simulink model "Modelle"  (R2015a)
settings: Solver=ode45  StartTime=0.0  StopTime=20  FixedStep=0.001  RelTol=1e-4
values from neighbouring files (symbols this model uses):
  A = [    [initLinear.m]    (also in Aufgabe_VglEigenwerte.m = initLinear( l, mp, ms, 0, 0, g, pi ); Versuch2.m = initLinear( l, mp, ms, 0, 0, g, pi ); linPendelZR.m = 1/n *     [ 0   n   0            0   ;                      ; linPendelZR2.m = [0, 1, 0, 0)
  AP = pi    (= 3.14159265359)    [Versuch1.m]    (also in Versuch2.m = 0; Versuch3.m = 0; simGUI.m = 0; Versuch4.m = 0)
  B = [0; 4; 0; 6/l]/(4*ms+mp)    [initLinear.m]    (also in linPendelZR.m = [0 a/n 0 b/n]'; linPendelZR2.m = [0)
  C = [1, 0, 0, 0    [initLinear.m]    (also in linPendelZR.m = [1 0 0 0; 0 0 1 0]')
  D = [0; 0]    [initLinear.m]    (also in linPendelZR.m = [0 0]')
  g = 9.81    [initModell.m]    (also in sFunModell.m = block.DialogPrm(6).Data; para.m; systemPendel_V3.m = stPendel.g; RandwertproblemDGL.m = stPendel.g)
  l = 0.41    [initModell.m]    (also in sFunModell.m = block.DialogPrm(5).Data; para.m; animierePendel.m = stPendel.lPendel; systemPendel_V3.m = stPendel.lPendel)
  mp = 0.177    [initModell.m]    (also in sFunModell.m = block.DialogPrm(3).Data; para.m; systemPendel_V3.m = stPendel.mPendel)
  ms = 7.055    [initModell.m]    (also in sFunModell.m = block.DialogPrm(1).Data; para.m; systemPendel_V3.m = stPendel.mSchlitten)
  Rp = 5.1e-3    (= 0.0051)    [initModell.m]    (also in sFunModell.m = block.DialogPrm(4).Data; para.m)
  Rs = 1.4    [initModell.m]    (also in sFunModell.m = block.DialogPrm(2).Data; para.m)
  teil = 1    [Versuch1.m]    (also in Versuch2.m = 4)
libraries: simulink x2

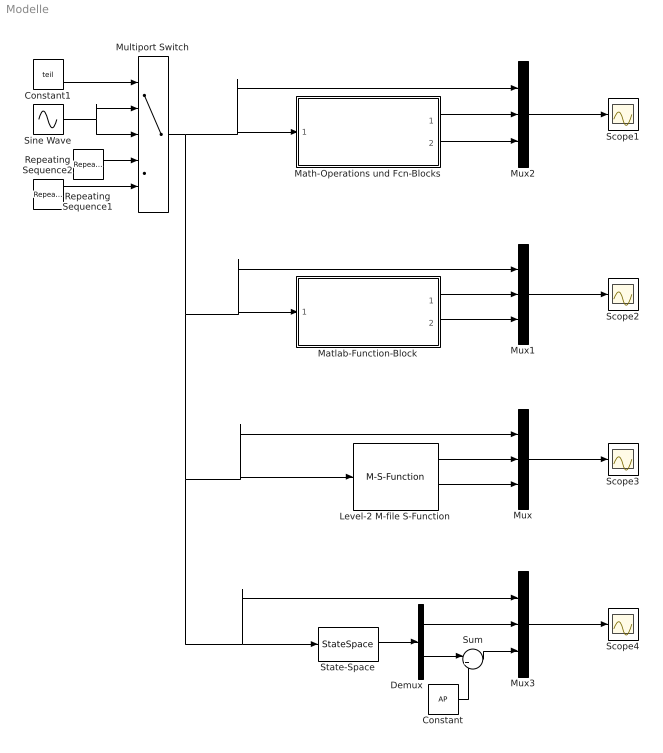
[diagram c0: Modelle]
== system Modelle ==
  Constant : Constant  Value=AP
  Constant1 : Constant  Value=teil
  Demux : Demux  Outputs=2
  Level-2 M-file S-Function : M-S-Function  FunctionName=sFunModell  Parameters=ms, Rs, mp, Rp, l, g, AP
  Math-Operations und Fcn-Blocks : Subsystem
  Matlab-Function-Block : Subsystem
  Multiport Switch : MultiPortSwitch  Inputs=4
  Mux{,1..3} (4 alike) : Mux  Inputs=3
  Repeating Sequence1 : simulink/Sources/Repeating Sequence  rep_seq_t=[0 0.5 0.5001 1.5 1.5001 2]  rep_seq_y=[40 40 -40 -40 40 40]
  Repeating Sequence2 : simulink/Sources/Repeating Sequence  rep_seq_t=[0 1 1.001 2 2.001]  rep_seq_y=[-40 -40 40 40 -40]
  Scope{1..4} (4 alike) : Scope
  Sine Wave : Sin  SampleTime=0
  State-Space : StateSpace  A=A  B=B  C=C  D=D  X0=[0 0 0 0]
  Sum : Sum  Inputs=|++
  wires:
  Math-Operations und Fcn-Blocks/1(xs) -> Mux2/2
  Math-Operations und Fcn-Blocks/2(phi) -> Mux2/3
  Matlab-Function-Block/1(xs) -> Mux1/2
  Matlab-Function-Block/2(phi) -> Mux1/3
  Level-2 M-file S-Function/1 -> Mux/2
  Level-2 M-file S-Function/2 -> Mux/3
  State-Space/1 -> Demux/1
  Demux/1 -> Mux3/2
  Multiport Switch/1 -> Level-2 M-file S-Function/1, Mux/1, Mux3/1, State-Space/1, Matlab-Function-Block/1(F), Mux1/1, Math-Operations und Fcn-Blocks/1(F), Mux2/1
  Mux2/1 -> Scope1/1
  Mux1/1 -> Scope2/1
  Mux3/1 -> Scope4/1
  Mux/1 -> Scope3/1
  Constant1/1 -> Multiport Switch/1
  Sine Wave/1 -> Multiport Switch/2, Multiport Switch/3
  Repeating Sequence1/1 -> Multiport Switch/4
  Repeating Sequence2/1 -> Multiport Switch/5
  Demux/2 -> Sum/1
  Sum/1 -> Mux3/3
  Constant/1 -> Sum/2

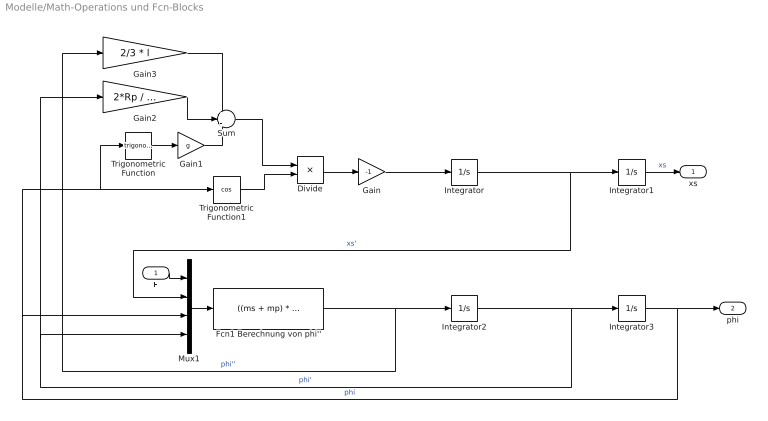
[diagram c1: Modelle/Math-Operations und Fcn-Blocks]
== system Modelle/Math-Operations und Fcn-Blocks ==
  F : Inport
  Divide : Product  Inputs=*/
  Fcn1 Berechnung von phi'' : Fcn  Expr=((ms + mp) * (g * sin(u(3)) + 2 * Rp/(mp*l) * u(4)) + mp * u(4)^2 * l/4 * sin(2*u(3)) + cos(u(3)) * (u(1) - Rs * u(2))) / (mp * l/2 * cos(u(3))^2 - (ms + mp) * 2/3 * l)
  Gain : Gain  Gain=-1
  Gain1 : Gain  Gain=g
  Gain2 : Gain  Gain=2*Rp / (mp*l)
  Gain3 : Gain  Gain=2/3 * l
  Integrator : Integrator
  Integrator1 : Integrator
  Integrator2 : Integrator
  Integrator3 : Integrator  InitialCondition=AP
  Mux1 : Mux
  Sum : Sum  Inputs=+++
  Trigonometric Function : Trigonometry
  Trigonometric Function1 : Trigonometry  Operator=cos
  xs : Outport
  phi : Outport  Port=2
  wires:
  Integrator/1 -> Integrator1/1, Mux1/2  "xs'"
  Integrator1/1 -> xs/1  "xs"
  Integrator2/1 -> Integrator3/1, Gain2/1, Mux1/4  "phi'"
  Integrator3/1 -> Trigonometric Function/1, Trigonometric Function1/1, Mux1/3, phi/1  "phi"
  Gain/1 -> Integrator/1
  Fcn1 Berechnung von phi''/1 -> Gain3/1, Integrator2/1  "phi''"
  Mux1/1 -> Fcn1 Berechnung von phi''/1
  F/1 -> Mux1/1
  Divide/1 -> Gain/1
  Trigonometric Function1/1 -> Divide/2
  Sum/1 -> Divide/1
  Gain1/1 -> Sum/3
  Trigonometric Function/1 -> Gain1/1
  Gain2/1 -> Sum/2
  Gain3/1 -> Sum/1

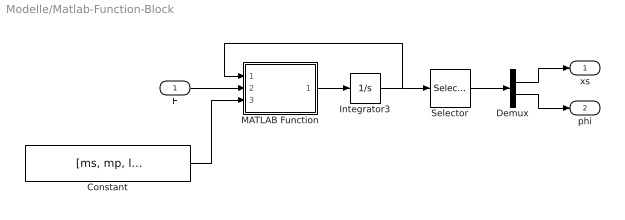
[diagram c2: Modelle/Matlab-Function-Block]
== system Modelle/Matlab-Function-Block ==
  F : Inport
  Constant : Constant  Value=[ms, mp, l, Rs, Rp, g]
  Demux : Demux  Outputs=2
  Integrator3 : Integrator  InitialCondition=[0; 0; AP; 0]
  MATLAB Function : MATLAB Function  TreatAsAtomicUnit=on
  Selector : Selector  InputPortWidth=4  IndexOptions=Index vector (dialog)  Indices=[1 3]  OutputSizes=1
  xs : Outport
  phi : Outport  Port=2
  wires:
  MATLAB Function/1(x_d) -> Integrator3/1
  Selector/1 -> Demux/1
  Demux/1 -> xs/1
  Integrator3/1 -> MATLAB Function/1(x), Selector/1
  Demux/2 -> phi/1
  F/1 -> MATLAB Function/2(F)
  Constant/1 -> MATLAB Function/3(p)

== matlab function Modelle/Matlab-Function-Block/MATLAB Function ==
function x_d  = fcn(x, F, p)
%#codegen

    %xs = x(1);
    xs_d = x(2);
    phi = x(3);
    phi_d = x(4);
    
    ms = p(1);
    mp = p(2);
    l = p(3);
    Rs = p(4);
    Rp = p(5);
    g = p(6);
    
	phi_dd = ( ...
                (ms + mp) * (g * sin(phi) + 2 * Rp/(mp*l) * phi_d) + ...
                    mp * phi_d^2 * l/4 * sin(2*phi) + ...
                    cos(phi) * (F - Rs * xs_d) ...
              ) / (mp * l/2 * cos(phi)^2 - (ms + mp) * 2/3 * l);
            
	xs_dd = -1/cos(phi) * ...
               (g * sin(phi) + 2 * Rp/(mp * l) * phi_d + 2/3 * l * phi_dd);
           
    x_d = [xs_d; xs_dd; phi_d; phi_dd];
